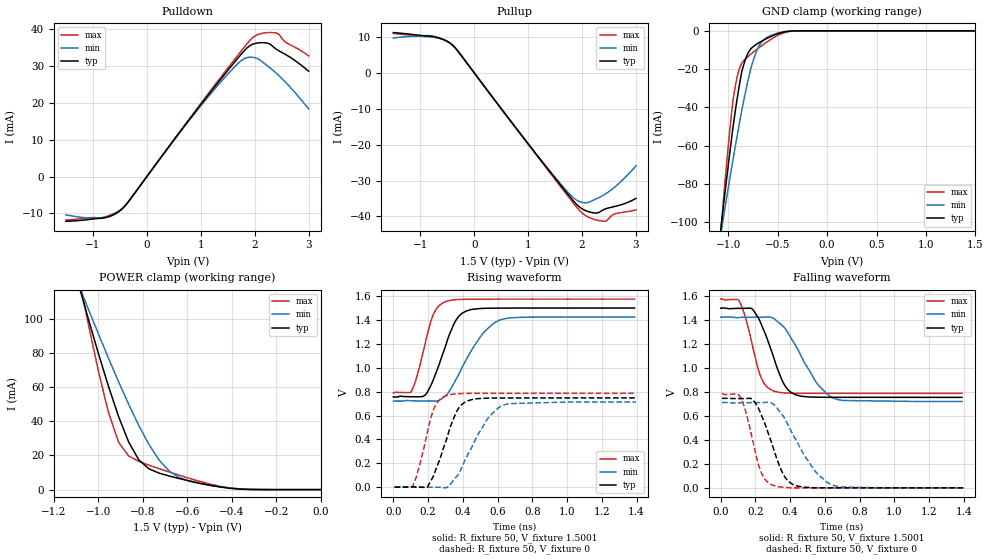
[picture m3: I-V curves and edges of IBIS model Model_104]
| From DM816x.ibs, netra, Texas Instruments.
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| Model based on original model for BSHTLTCSCDVGPBFZ
|   Sub model SLOW_8MA_5PER_1P5
[model]   Model_104
|[Description]  1.5V-3-STATE-X-SLOW, 8MA, +-5%
|[Input Load]
|[Output Drive] SLOW, 8MA
|Voltage   1.5V
|Mode   3-STATE
Model_type   3-state
Polarity   Non-Inverting
Enable   Active-Low
Cref =  15.0000pF
Rref =  100.0000M
Vref =  0V
Vmeas =  0.75005
C_comp   1.5249p   1.4275p   1.6205p
[Model Spec]
[Temperature Range]   25   125   -40
[Voltage Range]   1.5   1.425   1.575
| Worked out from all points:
|   slope of the pulldown table from 0 to 0.225 V, typ, clamps not added: 50.1 ohm
|   slope of the pullup table from 0 to 0.225 V, typ, clamps not added: 50.1 ohm
|   GND clamp passes 1 mA (typ) near -0.47 V on its own axis
|   POWER clamp passes 1 mA (typ) near -0.42 V on its own axis
|   rising waveform, R_fixture 50, V_fixture 1.5001: 20-80 % time 112ps typ, 168ps min, 83.2ps max; typ from 0.756 V to 1.5 V
|   rising waveform, R_fixture 50, V_fixture 0: 20-80 % time 108ps typ, 154ps min, 80.3ps max; typ from 0 V to 0.747 V
|   falling waveform, R_fixture 50, V_fixture 1.5001: 20-80 % time 114ps typ, 168ps min, 82.8ps max; typ from 1.5 V to 0.755 V
|   falling waveform, R_fixture 50, V_fixture 0: 20-80 % time 111ps typ, 170ps min, 80.3ps max; typ from 0.746 V to 0 V
[POWER_clamp]
-1.5V     321.7mA    260.6mA    415.9mA
-1.076V   114.2mA    115.8mA    116.9mA
-1.061V   107.2mA    110.9mA    107.1mA
-954.6mV  60.59mA    77.06mA    45.35mA
-909.2mV  42.85mA    63.21mA    27.81mA
-863.7mV  27.9mA     49.99mA    19.69mA
-818.2mV  17.49mA    37.63mA    16.52mA
-772.8mV  12.19mA    26.53mA    14.33mA
-681.9mV  7.985mA    10.89mA    10.33mA
-590.9mV  5.094mA    4.955mA    6.6mA
-363.7mV  298.5uA    465.2uA    297.6uA
0V        1.518nA    24.08nA    367.8pA
[Pulldown]
-1.5V     -12.15mA   -10.4mA    -11.83mA
-863.7mV  -11.34mA   -11.22mA   -11.25mA
-500mV    -9.267mA   -9.352mA   -9.148mA
-318.2mV  -6.354mA   -6.371mA   -6.385mA
1.046V    20.42mA    20.05mA    20.72mA
1.591V    30.47mA    29.26mA    31.18mA
1.818V    34.39mA    32.13mA    35.4mA
1.955V    35.92mA    32.45mA    37.67mA
2.091V    36.38mA    31.76mA    38.77mA
2.273V    36.08mA    29.69mA    39.15mA
2.364V    35.03mA    28.59mA    39.11mA
3V        28.64mA    18.41mA    32.82mA
[Pullup]
-1.5V     11.21mA    9.69mA     10.94mA
-818.2mV  10.23mA    9.978mA    10.29mA
-590.9mV  9.401mA    9.328mA    9.374mA
-409.1mV  7.828mA    7.781mA    7.859mA
1.227V    -24.14mA   -24.11mA   -24.35mA
1.727V    -33.63mA   -33.09mA   -34.13mA
1.909V    -36.81mA   -35.55mA   -37.6mA
2.046V    -38.25mA   -36.2mA    -39.57mA
2.227V    -39.04mA   -35.36mA   -40.83mA
2.409V    -38.05mA   -33.98mA   -41.36mA
2.591V    -37.29mA   -32.03mA   -39.38mA
3V        -34.98mA   -25.95mA   -38.2mA
[GND_clamp]
-1.5V     -310.1mA   -250.5mA   -402.5mA
-1.076V   -103.6mA   -106.2mA   -105.2mA
-1.046V   -89.81mA   -96.36mA   -86.02mA
-954.6mV  -51.22mA   -67.87mA   -36.88mA
-924.3mV  -40.08mA   -58.86mA   -27.29mA
-863.7mV  -21.24mA   -41.56mA   -16.73mA
-833.4mV  -15.8mA    -33.75mA   -15.03mA
-772.8mV  -9.345mA   -19.75mA   -12.19mA
-712.2mV  -6.928mA   -10.35mA   -9.704mA
-621.3mV  -4.261mA   -3.896mA   -6.225mA
-409.1mV  -337.1uA   -289.1uA   -618.9uA
1.5V      1.518nA    257.2nA    299pA
[Ramp]
dV/dt_f   0.596016/0.16747067n   0.56408/0.25220681n   0.629272/0.12664996n
dV/dt_r 0.60150488/0.15902866n  0.5749704/0.2367164n  0.6310776/0.12226898n
R_load = 50
[Rising Waveform]
R_fixture = 50
V_fixture = 1.5001
V_fixture_min = 1.425
V_fixture_max = 1.575
0s        755.9mV    721.1mV    789.3mV
105.6ps   757.6mV    723.4mV    805.5mV
190.6ps   784mV      722.2mV    1.249V
234.2ps   914.3mV    721.9mV    1.459V
291.2ps   1.142V     755.2mV    1.548V
350.6ps   1.371V     876mV      1.569V
396.4ps   1.457V     1.003V     1.573V
510.7ps   1.497V     1.279V     1.575V
605.1ps   1.5V       1.395V     1.575V
1.389ns   1.5V       1.425V     1.575V
[Rising Waveform]
R_fixture = 50
V_fixture = 0
V_fixture_min = 0
V_fixture_max = 0
7.64ps    0V         0V         0V
112.5ps   2.402mV    2.288mV    11.38mV
196.4ps   4.593mV    0V         463.9mV
237.2ps   116mV      0V         668.8mV
297.3ps   362.9mV    -5.868mV   761.9mV
355.8ps   605.8mV    76.01mV    780.7mV
400.8ps   700.1mV    187.9mV    784.3mV
536.5ps   745.2mV    560.4mV    786.1mV
626.9ps   746.9mV    683.6mV    786.2mV
1.397ns   747.3mV    712.8mV    786.3mV
[Falling Waveform]
R_fixture = 50
V_fixture = 1.5001
V_fixture_min = 1.425
V_fixture_max = 1.575
0s        1.499V     1.424V     1.575V
106.7ps   1.498V     1.421V     1.558V
179.4ps   1.494V     1.424V     1.209V
227.6ps   1.385V     1.423V     938.4mV
309.5ps   1.069V     1.408V     806mV
361.2ps   874.6mV    1.346V     793.1mV
409.7ps   792.2mV    1.238V     790mV
552.7ps   756.4mV    875mV      788.7mV
651.7ps   755.4mV    747.4mV    788.6mV
1.389ns   755.2mV    720.6mV    788.5mV
[Falling Waveform]
R_fixture = 50
V_fixture = 0
V_fixture_min = 0
V_fixture_max = 0
7.64ps    746.4mV    711.9mV    785.4mV
114.6ps   744.5mV    709.9mV    754.8mV
183.1ps   737mV      711.7mV    403.9mV
235.7ps   602.7mV    711.3mV    120.3mV
307.2ps   313.1mV    693.7mV    17.79mV
359.3ps   116.2mV    599.2mV    4.726mV
404.2ps   38.42mV    476.5mV    0V
536.5ps   0V         153.6mV    0V
626.6ps   0V         34.67mV    0V
1.397ns   0V         0V         0V
